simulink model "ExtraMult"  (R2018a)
settings: Solver=VariableStepAuto  StartTime=0.0  StopTime=30  RelTol=1e-3
undefined symbols (not defined in the file): a091, d685b336cacf, ExtraMult, sdiscope

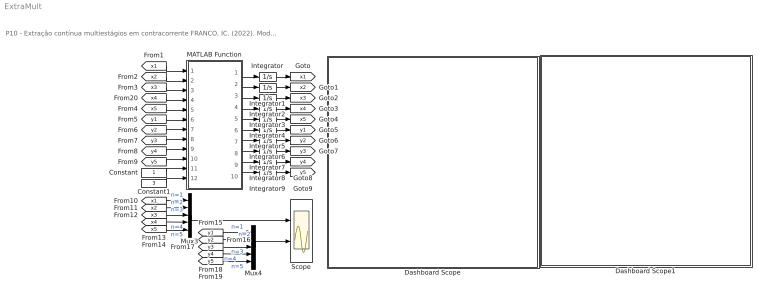
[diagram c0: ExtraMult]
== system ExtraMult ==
  note: P10 - Extração contínua multiestágios em contracorrente FRANCO, IC. (2022). Modelagem e Simulação: Problemas Típicos da Engenharia Química para Simulação e Análise. NOTAS DE AULA INOVADORAS. The Journal of Engineering and Exact Sciences. Material Complementar.
  Constant : Constant
  Constant1 : Constant  Value=3
  Dashboard Scope : Subsystem  DialogController=hmiCreateDDGDialog  IsWebBlock=on  mask(MWDashboardBlock){webBlockId=59d600c1-e791-4fa7-a091-312a2da81686, webBlockType=sdiscope, ShowInitialText=on, HMISrcModelName=ExtraMult}
      mask prompts: webBlockId "WebBlock Id"; webBlockType "WebBlock Type"; HMISrcModelName "Source Model"
      mask help: SimulinkHMI:dialogs:HMIScopeDialogDesc
  Dashboard Scope1 : Subsystem  DialogController=hmiCreateDDGDialog  IsWebBlock=on  mask(MWDashboardBlock){webBlockId=7625b0fe-33d2-4171-86e9-d685b336cacf, webBlockType=sdiscope, ShowInitialText=on, HMISrcModelName=ExtraMult}
      mask prompts: webBlockId "WebBlock Id"; webBlockType "WebBlock Type"; HMISrcModelName "Source Model"
      mask help: SimulinkHMI:dialogs:HMIScopeDialogDesc
  Integrator{,1..9} (10 alike) : Integrator
  MATLAB Function : MATLAB Function  TreatAsAtomicUnit=on
  Mux3 : Mux  Inputs=5
  Mux4 : Mux  Inputs=5
  Scope : Scope  NumInputPorts=2
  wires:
  [y4] -> MATLAB Function/9(y4)
  Integrator5/1 -> [y1]
  Integrator3/1 -> [x4]
  Constant1/1 -> MATLAB Function/12(G)
  [y1] -> MATLAB Function/6(y1)
  Constant/1 -> MATLAB Function/11(L)
  [y3] -> MATLAB Function/8(y3)
  MATLAB Function/4(dx4) -> Integrator3/1
  Integrator8/1 -> [y4]
  MATLAB Function/10(dy5) -> Integrator9/1
  MATLAB Function/5(dx5) -> Integrator4/1
  [x5] -> MATLAB Function/5(x5)
  [y5] -> MATLAB Function/10(y5)
  MATLAB Function/9(dy4) -> Integrator8/1
  [y2] -> MATLAB Function/7(y2)
  MATLAB Function/2(dx2) -> Integrator1/1
  MATLAB Function/8(dy3) -> Integrator7/1
  Integrator4/1 -> [x5]
  MATLAB Function/3(dx3) -> Integrator2/1
  Integrator/1 -> [x1]
  Integrator2/1 -> [x3]
  Integrator7/1 -> [y3]
  Integrator9/1 -> [y5]
  Integrator6/1 -> [y2]
  Integrator1/1 -> [x2]
  MATLAB Function/6(dy1) -> Integrator5/1
  MATLAB Function/7(dy2) -> Integrator6/1
  MATLAB Function/1(dx1) -> Integrator/1
  Mux4/1 -> Scope/2
  [y1] -> Mux4/1  "n=1"
  [y3] -> Mux4/3  "n=3"
  [y5] -> Mux4/5  "n=5"
  [x3] -> Mux3/3  "n=3"
  [x1] -> Mux3/1  "n=1"
  Mux3/1 -> Scope/1
  [x5] -> Mux3/5  "n=5"
  [y4] -> Mux4/4  "n=4"
  [x4] -> Mux3/4  "n=4"
  [y2] -> Mux4/2  "n=2"
  [x2] -> Mux3/2  "n=2"
  [x1] -> MATLAB Function/1(x1)
  [x2] -> MATLAB Function/2(x2)
  [x3] -> MATLAB Function/3(x3)
  [x4] -> MATLAB Function/4(x4)

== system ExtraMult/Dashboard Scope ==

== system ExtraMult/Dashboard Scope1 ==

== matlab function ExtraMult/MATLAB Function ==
function [dx1,dx2,dx3,dx4,dx5,dy1,dy2,dy3,dy4,dy5] = fcn(x1,x2,x3,x4,x5,y1,y2,y3,y4,y5,L,G)
% Parâmetros
k   = 50.00;
Keq =  0.80;
Vx  =  2.00;
Vy  =  2.00;
x0  =  1.00;
y6  =  0.00;

%% equações auxiliares
% taxa de transferência de massa
Q1=k*(x1-y1/Keq);
Q2=k*(x2-y2/Keq);
Q3=k*(x3-y3/Keq);
Q4=k*(x4-y4/Keq);
Q5=k*(x5-y5/Keq);
    
%% Modelo matemático
dx1 = (L*(x0-x1)-Q1)/Vx;
dx2 = (L*(x1-x2)-Q2)/Vx;
dx3 = (L*(x2-x3)-Q3)/Vx;
dx4 = (L*(x3-x4)-Q4)/Vx;
dx5 = (L*(x4-x5)-Q5)/Vx;

dy1 = (G*(y2-y1)+Q1)/Vy;
dy2 = (G*(y3-y2)+Q2)/Vy;
dy3 = (G*(y4-y3)+Q3)/Vy;
dy4 = (G*(y5-y4)+Q4)/Vy;
dy5 = (G*(y6-y5)+Q5)/Vy;
end
